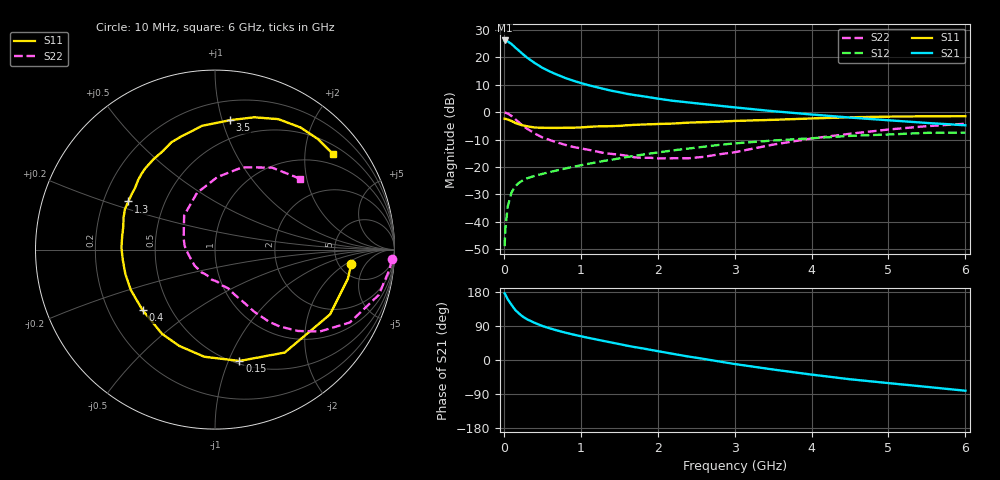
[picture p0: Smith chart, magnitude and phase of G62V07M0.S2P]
! SIEMENS Small Signal Semiconductors
! BFG193
! Si NPN RF Bipolar Junction Transistor in SOT223
! VCE = 2 V  IC = 7 mA
! Common Emitter S-Parameters:  August  1996
# GHz  S  MA  R  50
!  f  S11  S21  S12  S22
! GHz  MAG  ANG  MAG  ANG  MAG  ANG  MAG  ANG
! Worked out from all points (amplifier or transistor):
!   36 points, 10 MHz to 6 GHz, reference 50 ohm
!   highest |S21| = 26.2 dB at 10 MHz (marker M1)
!   |S21| within 3 dB of that: start of sweep to 166.1 MHz
!   unconditionally stable (mu >= 1): 974.4 MHz to 2.685 GHz
!   at 250 MHz: K = 0.43, MSG = 23.0 dB, |S12| = -24.8 dB
!   at 1.4 GHz: K = 1.08, MAG = 10.8 dB, |S12| = -17.3 dB
!   at 6 GHz: K = 0.91, MSG = 1.3 dB, |S12| = -7.4 dB
!   S11 on the Smith chart (normalised r, x): 10 MHz: 6.53, -2.46; 150 MHz: 0.53, -1.10; 400 MHz: 0.35, -0.32; 1.3 GHz: 0.31, +0.24; 3.5 GHz: 0.35, +1.06; 6 GHz: 0.71, +2.67
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0.01  0.7641 -5.9  20.36 176.0  0.0036 89.0  0.9859 -3.2
0.02  0.7578 -12.4  20.27 172.8  0.0075 83.2  0.9796 -6.3
0.05  0.7356 -29.4  19.54 160.5  0.0189 74.7  0.9464 -15.5
0.1  0.6928 -55.9  17.56 145.5  0.0344 65.3  0.854 -28.4
0.15  0.6352 -77.6  15.07 131.6  0.045 55.9  0.7403 -38.1
0.2  0.5999 -95.7  13.12 122.2  0.052 50.9  0.6468 -44.5
0.25  0.5725 -110.3  11.36 114.0  0.0576 47.4  0.5614 -49.8
0.3  0.5547 -122.1  9.951 107.7  0.062 45.2  0.5037 -53.1
0.4  0.5259 -140.1  7.913 98.1  0.0689 43.0  0.41 -57.7
0.5  0.5203 -154.3  6.474 89.8  0.0749 42.0  0.3478 -60.6
0.6  0.5176 -164.6  5.511 83.4  0.0812 42.1  0.3096 -63.2
0.7  0.517 -173.4  4.788 77.5  0.0873 42.4  0.2794 -65.9
0.9  0.5224 172.2  3.765 67.3  0.1007 42.2  0.233 -70.3
1.1  0.5403 160.5  3.114 58.4  0.1145 42.1  0.2061 -77.9
1.3  0.5519 150.9  2.655 50.1  0.1292 41.1  0.1803 -85.3
1.6  0.5775 137.9  2.164 37.8  0.1521 38.0  0.1603 -101.1
2.2  0.6208 117.9  1.614 16.2  0.2011 29.7  0.1445 -141.6
2.8  0.6734 100.8  1.312 -3.9  0.2533 18.7  0.1707 172.8
3.5  0.7258 83.4  1.044 -25.1  0.3045 2.9  0.2564 132.1
4.5  0.808 64.1  0.798 -50.8  0.3699 -16.8  0.4046 88.1
5.5  0.8418 47.0  0.637 -70.9  0.4202 -41.0  0.5567 55.1
6  0.8464 38.8  0.577 -81.1  0.4243 -54.9  0.6159 39.9
